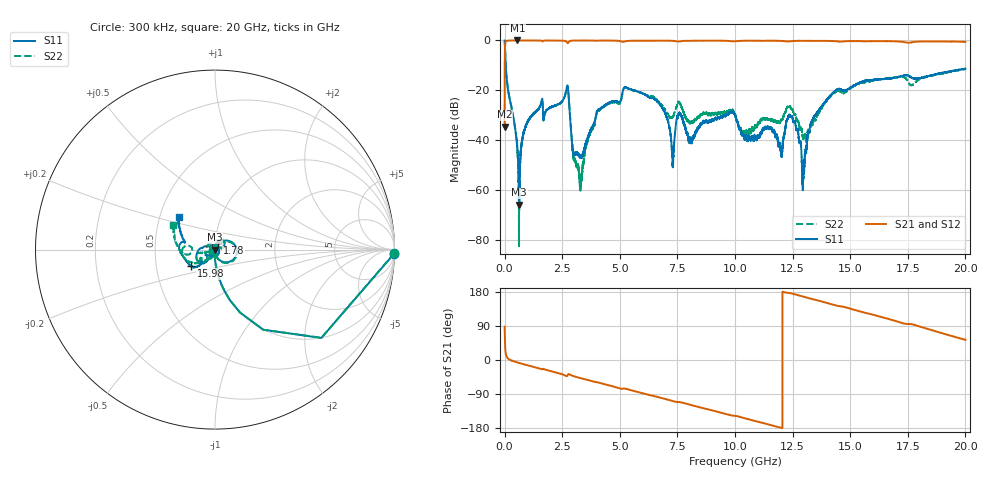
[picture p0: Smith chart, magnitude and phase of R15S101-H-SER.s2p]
!{R15S101}
!Johanson Technology Inc.
!www.johansontechnology.com
!Test Board Conditions:
!Substrate Type  RO4350B
!Substrate Thickness  20 mil
!Substrate Dk  3.66
!TL Type: GCPW
!TL Trace Width  34 mil
!TL Gap  10 mil
!Electrode orientation  Horizontal
!DUT TOPOLOGY	SERIES
!Mounting Pad LxW  26x52 mil
! Created Sat Feb  6 14:05:51 2021
# hz S ma R 50
! 2 Port Network Data from SP1.SP block
! freq  magS11  angS11  magS21  angS21  magS12  angS12  magS22  angS22
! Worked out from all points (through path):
!   20001 points, 300 kHz to 20 GHz, reference 50 ohm
!   highest |S21| = 0.00 dB at 557.3 MHz (marker M1); lowest = -34.6 dB at 300 kHz (marker M2)
!   group delay of S21, straight-line fit = 42.5 ps
!   lowest |S11| = -65.8 dB at 635.3 MHz (marker M3), VSWR 1.00, Z = 50 + j0.0355 ohm
!   |S11| at or under -10 dB: 47.94 MHz to end of sweep
!   |S22| runs from -82.4 to 0.0 dB; largest |S21 - S12| = 0.014
!   S11 on the Smith chart (normalised r, x): 300 kHz: 5, -87; 1.78 GHz: 1.03, +0.07; 15.98 GHz: 0.75, -0.14; 20 GHz: 0.63, +0.25
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300000  0.9986 -1.3  0.01869 88.1  0.01867 88.8  0.9982 -1.2
1.093e8  0.1425 -83.1  0.989 6.8  0.9895 6.7  0.1432 -83.2
5.573e8  0.006414 -99.7  1 -6.6  0.9992 -6.6  0.006362 -95.7
6.353e8  0.0005148 136.3  0.9998 -8.0  0.9994 -8.0  0.0007485 94.3
1.0023e9  0.02323 79.9  0.9989 -14.1  0.9988 -14.1  0.02383 75.8
1.7803e9  0.03761 67.7  0.997 -25.6  0.997 -25.6  0.03722 56.8
2.7063e9  0.118 7.6  0.9157 -42.8  0.915 -42.8  0.1197 4.3
2.9913e9  0.005191 -28.4  0.9931 -42.5  0.993 -42.5  0.004637 -42.1
3.3343e9  0.004534 -39.7  0.9971 -48.4  0.9966 -48.4  0.001664 120.6
4.1083e9  0.04171 -131.6  0.9931 -60.2  0.9932 -60.1  0.03987 -159.3
6.6673e9  0.05767 161.2  0.99 -97.9  0.9905 -97.9  0.05998 -168.0
7.2933e9  0.003583 -176.3  0.9815 -108.3  0.9816 -108.3  0.02861 -117.8
7.5713e9  0.03508 -145.0  0.9529 -110.9  0.9539 -111.0  0.05827 -128.9
8.0683e9  0.01006 76.0  0.9894 -118.3  0.9887 -118.3  0.02335 -112.3
1.00003e10  0.03281 -142.1  0.9615 -147.3  0.9611 -147.3  0.03365 -151.4
1.19783e10  0.006519 116.8  0.9797 -178.6  0.9803 -178.7  0.02429 151.4
1.24153e10  0.02938 123.7  0.9656 176.2  0.9637 176.2  0.04382 136.1
1.29773e10  0.00212 143.9  0.9857 167.0  0.9859 167.0  0.01085 139.0
1.33343e10  0.02362 -116.9  0.9822 161.2  0.9818 161.1  0.02141 -137.9
1.59763e10  0.1619 -145.9  0.9657 119.7  0.9683 119.6  0.1557 -153.8
1.66673e10  0.1707 -158.8  0.9669 108.1  0.9567 108.1  0.1777 -164.1
2e10  0.2684 137.0  0.9373 53.1  0.9288 52.9  0.2724 149.0
